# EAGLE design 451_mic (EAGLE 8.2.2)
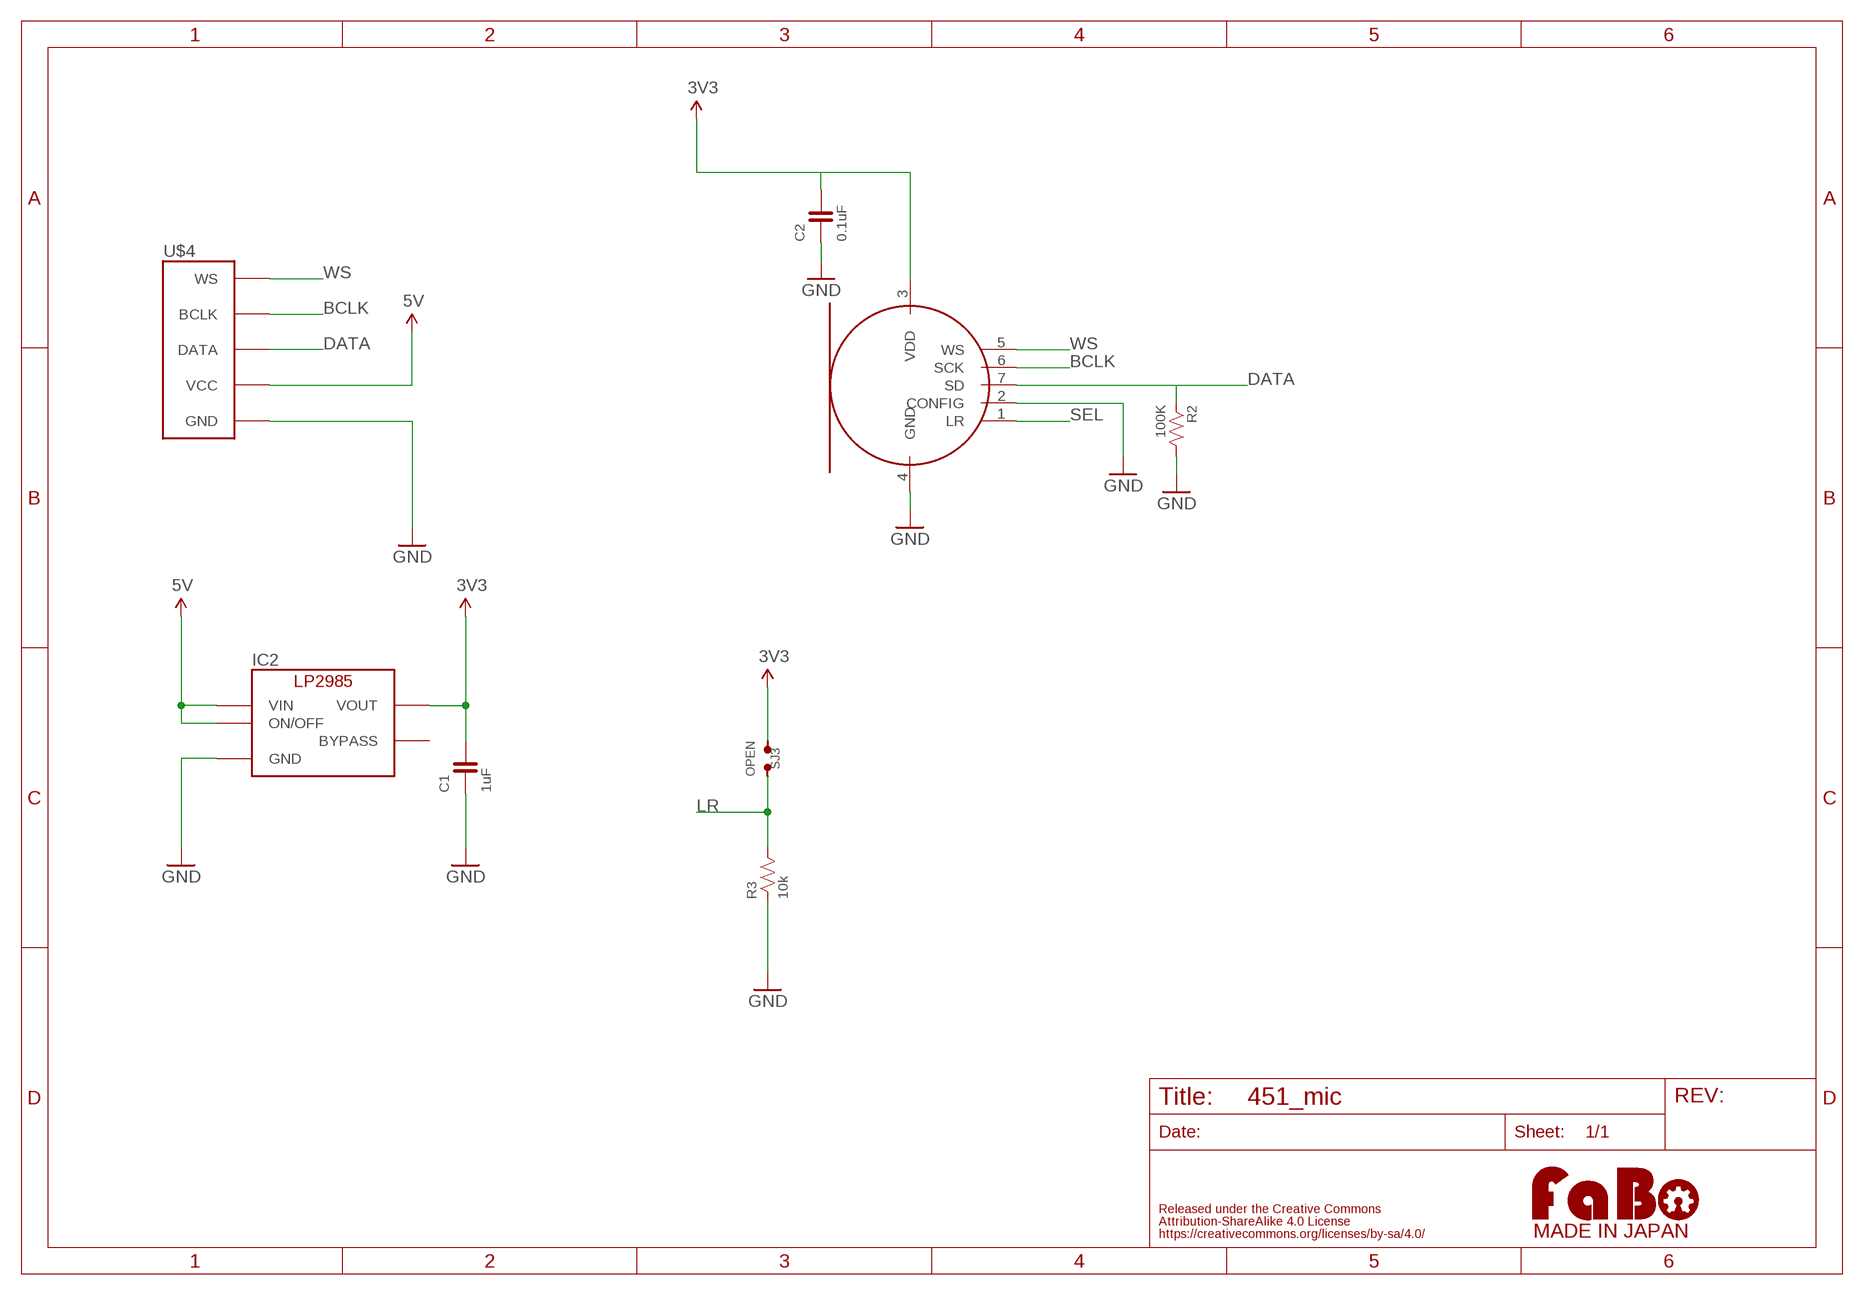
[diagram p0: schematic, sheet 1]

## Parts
C1  1uF  CAPACITOR-0603  [0603]
C2  0.1uF  CAPACITOR-0603  [0603]
IC2  LP2985-33DBV  [SOT-23-5]
MIC  TDK-ICS43432  [TDK-ICS43432]
R2  100K  RESISTOR-0603  [0603]
R3  10k  RESISTOR-0603  [0603]
SJ3  OPEN  SMD-JUMPER-2-OPEN  [SMD-JUMPER-2-OPEN]
U$3  LOGO_FABO-M_BOTTOM  [LOGO_FABO_MS_BOTTOM]
U$4  FABO_BRICK_I2S  [FABO_BRICK_I2S]

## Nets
3V3: C1.2 C2.2 IC2.5(VOUT) MIC.3(VDD) SJ3.1
5V: IC2.1(VIN) IC2.3(ON/OFF) U$4.VCC
BCLK: MIC.6(SCK) U$4.BCLK
DATA: MIC.7(SD) R2.1 U$4.DATA
GND: C1.1 C2.1 IC2.2(GND) MIC.2(CONFIG) MIC.4(GND) R2.2 R3.1 U$4.GND
LR: R3.2 SJ3.2
SEL: MIC.1(LR)
WS: MIC.5(WS) U$4.WS
Unconnected: IC2.4(BYPASS)

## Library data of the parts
C1 C2 = FaBo-Capacitor:CAPACITOR: CAPACITOR
IC2 = FaBo-Supply:LP2985: LP2985
MIC = FaBo-Mems:TDK-ICS43432
R2 R3 = FaBo-Resistors:RESISTOR: RESISTOR
SJ3 = FaBo-Supply:SMD-JUMPER-2
U$3 = FaBo-etc:LOGO_FABO
U$4 = FaBo-Template:FABO_BRICK_I2S

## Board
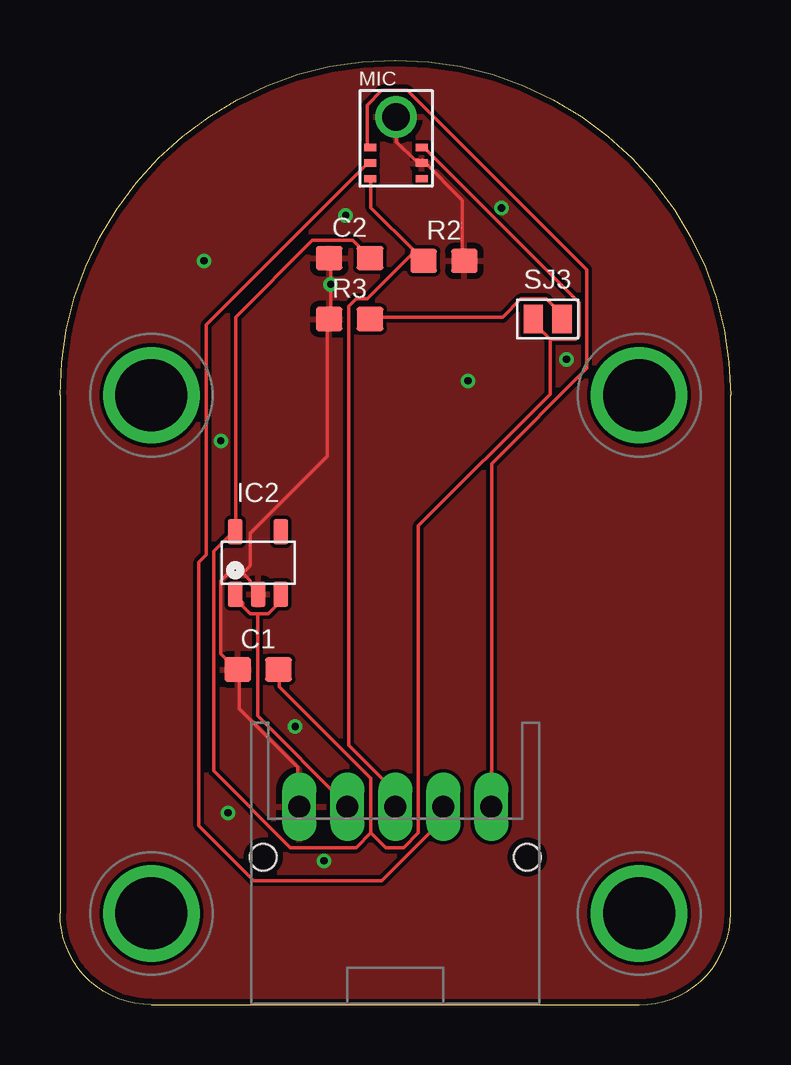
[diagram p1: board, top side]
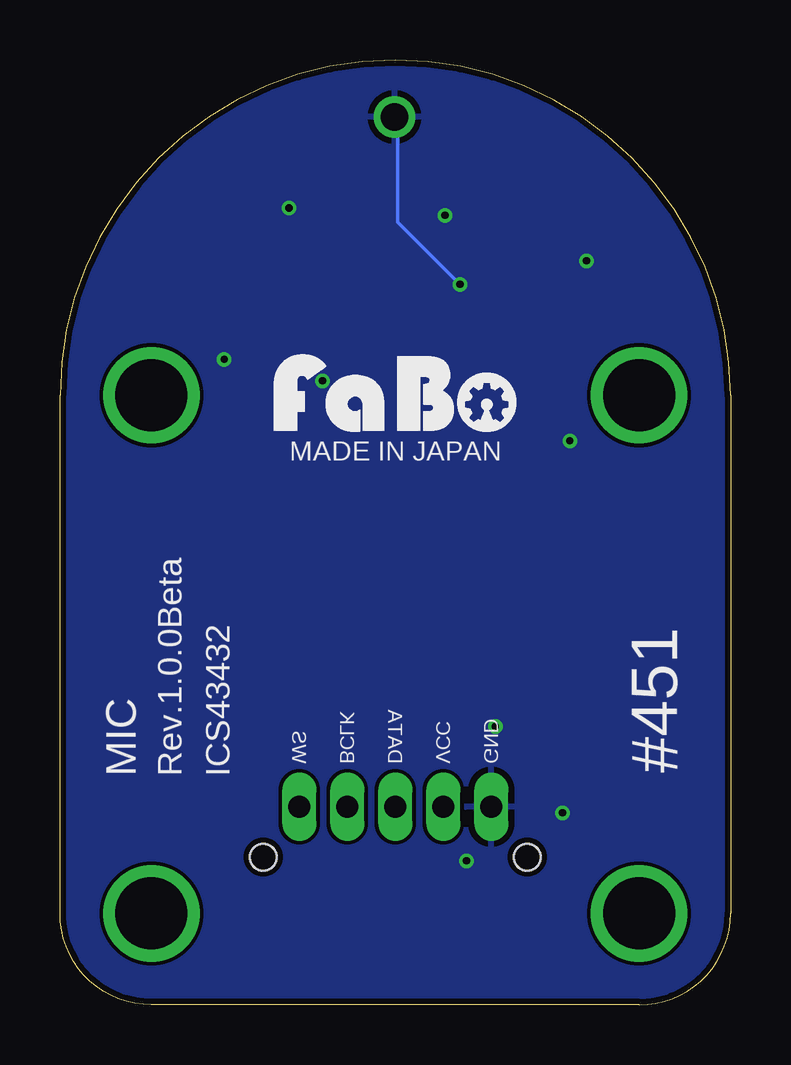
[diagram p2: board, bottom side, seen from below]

Size 27.94 x 39.37 mm. Coordinates in mm from the lower left corner, seen from the top.
Copper layers (1*16): Top 0.035mm / dielectric 1.5mm / Bottom 0.035mm
Design rules "Elecrow_angle": minimum track width 6mil, minimum drill 12mil, track to track 6mil, track to pad 6mil, pad to pad 6mil, via to via 6mil, smd to smd 0mil, copper to edge 10mil, drill to drill 10mil, minimum pad ring 10mil, minimum via ring 6mil, stop-mask expansion 2mil, vias tented up to drill 100mil, thermal gap 10mil

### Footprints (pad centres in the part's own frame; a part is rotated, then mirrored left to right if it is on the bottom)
0603 = smd 1.1 x 1: 1 -0.85,0; 2 0.85,0
SOT-23-5 = smd 0.6 x 1.05: 1 -0.95,-1.3; 2 0,-1.3; 3 0.95,-1.3; 4 0.95,1.3; 5 -0.95,1.3
TDK-ICS43432 = smd 0.5 x 0.3: 1 1.075,-2.575; 2 1.075,-1.925; 3 1.075,-1.275; 5 -1.075,-1.275; 6 -1.075,-1.925; 7 -1.075,-2.575 | drill 1.15 pad 1.65: 4 0,0
SMD-JUMPER-2-OPEN = smd 0.8 x 1.2: 1 -0.6,0; 2 0.6,0
FABO_BRICK_I2S = drill 0.9 pad 1.422 long: BCLK 2,-9.525; DATA 0,-9.525; GND -4,-9.525; VCC -2,-9.525; WS 4,-9.525 | drill 3 pad 3.81: P$1 -10.16,7.62; P$2 10.16,7.62; P$3 -10.16,-13.97; P$4 10.16,-13.97 | hole 1.1: -5.5,-11.625; 5.5,-11.625

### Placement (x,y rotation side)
C1  8.26,13.97 0 top
C2  12.06,31.11 0 top
IC2  8.26,18.41 0 top
MIC  14,37 0 top
R2  16,31 0 top
R3  12.06,28.57 0 top
SJ3  20.32,28.57 0 top
U$3  13.97,23.5 0 top
U$4  13.97,17.78 0 top

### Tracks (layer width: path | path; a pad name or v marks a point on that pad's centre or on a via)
3V3
  Top 0.152: 20.42,27.74 21.49,27.74 21.64,27.89 21.64,29.26 15.24,35.66 15.09,35.66 MIC.3 | 20.42,27.74 19.66,28.5 SJ3.1 | C2.2 12.8,31.24 12.19,31.85 10.52,31.85 7.32,28.65 7.32,19.81 IC2.5 7.16,19.66 6.4,18.9 6.4,9.75 9.6,6.55 12.34,6.55 12.95,7.16 | 12.95,7.16 12.95,9.45 9.14,13.26 9.14,13.87 C1.2 | 20.42,27.74 20.42,25.45 14.94,19.96 14.94,7.16 14.33,6.55 13.56,6.55 12.95,7.16
5V
  Top 0.152: 8.23,16.31 8.69,16.31 9.14,16.76 9.14,17.07 IC2.3 | 8.23,16.31 7.92,16.31 7.62,16.61 7.62,16.76 7.32,17.07 IC2.1 | 8.23,16.31 8.23,12.04 11.89,8.38 U$4.VCC
BCLK
  Top 0.152: MIC.6 12.8,35.05 6.1,28.35 6.1,18.75 5.79,18.44 5.79,7.47 8.08,5.18 13.41,5.18 15.85,7.62 15.85,8.23 U$4.BCLK
DATA
  Top 0.152: 14.78,31.39 15.09,31.09 R2.1 14.78,31.39 | 14.78,31.39 12.95,33.22 12.95,34.29 MIC.7 | 14.78,31.39 12.8,29.41 12.34,29.41 12.04,29.11 12.04,10.82 13.87,8.99 13.87,8.38 U$4.DATA
GND  (via drill 0.3)
  Top 0.152: MIC.4 14.02,36.88 14.02,35.97 14.78,35.2 14.94,35.2 MIC.2 15.09,35.2 16.76,33.53 16.76,31.09 R2.2 | C2.1 11.28,31.09 v11.28,30.02 11.28,28.65 R3.1 11.12,28.5 11.12,22.86 7.92,19.66 7.92,18.29 7.62,17.98 | 7.62,17.98 7.92,17.68 7.92,17.53 8.23,17.22 IC2.2 | 7.62,17.98 7.01,17.98 6.71,17.68 6.71,14.63 7.32,14.02 C1.1 7.47,13.87 7.47,12.34 9.91,9.91 9.91,8.38 U$4.GND
  Bottom 0.152: v11.28,30.02 13.87,32.61 13.87,36.88 MIC.4
  other vias: 6,31 17,26 7,8 11,6 9.8,11.6 6.7,23.5 21.1,26.9 11.9,32.9 18.4,33.2
  pour Bottom: 0,0 28,0 28,40 0,40
  pour Top: 0,0 28,0 28,40 0,40
LR
  Top 0.152: R3.2 12.95,28.65 18.44,28.65 19.2,29.41 20.27,29.41 21.03,28.65 SJ3.2
WS
  Top 0.152: MIC.5 12.8,35.81 12.8,37.49 13.41,38.1 14.48,38.1 21.95,30.63 21.95,26.52 17.98,22.55 17.98,8.38 U$4.WS

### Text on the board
bPlace: MADE IN JAPAN | #451 | ICS43432 | Rev.1.0.0Beta | MIC

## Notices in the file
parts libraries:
FaBo-etc: Released under the Creative Commons Attribution-ShareAlike 4.0 License
https://creativecommons.org/licenses/by-sa/4.0
FaBo-etc: Released under the Creative Commons
